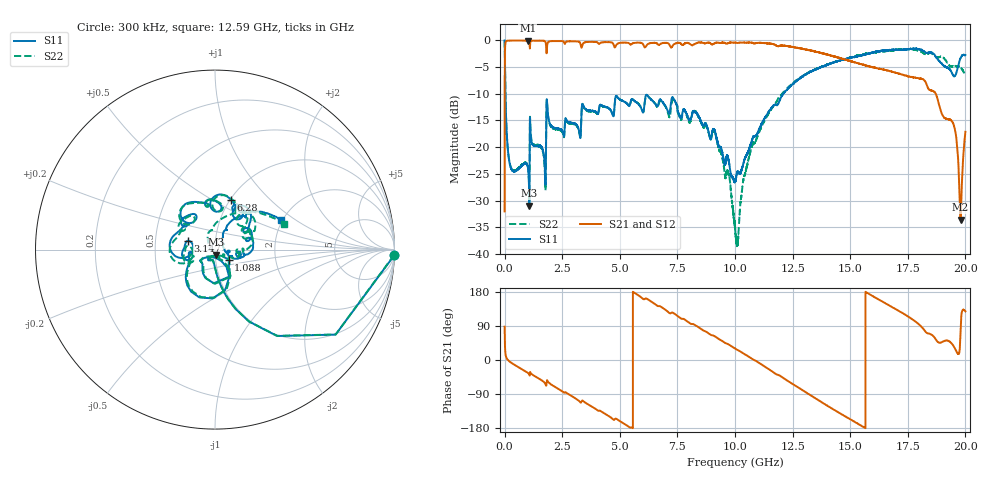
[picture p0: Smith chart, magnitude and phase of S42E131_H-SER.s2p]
! Created Wed Nov 25 21:58:57 2020
# khz S ma R 50
! 2 Port Network Data from SP1.SP block
! freq  magS11  angS11  magS21  angS21  magS12  angS12  magS22  angS22
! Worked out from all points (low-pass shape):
!   20001 points, 300 kHz to 20 GHz, reference 50 ohm
!   highest |S21| = -0.02 dB at 1.005 GHz (marker M1); lowest = -33.6 dB at 19.79 GHz (marker M2)
!   |S21| within 3 dB of the highest: 12.05 MHz to 14.32 GHz (14.3 GHz wide, 200 % of centre); 14.31797 GHz to 14.31964 GHz (1.671 MHz wide, 0.0117 % of centre)
!   lowest |S11| = -31.0 dB at 1.074 GHz (marker M3), VSWR 1.06, Z = 50.4 - j2.82 ohm
!   |S11| at or under -10 dB: 36.14 MHz to 12.1 GHz (12.06 GHz wide, 199 % of centre)
!   |S22| runs from -38.5 to 0.0 dB; largest |S21 - S12| = 0.017
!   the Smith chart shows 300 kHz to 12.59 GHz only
!   S11 on the Smith chart (normalised r, x): 300 kHz: 3, -61; 1.088 GHz: 1.16, -0.13; 3.147 GHz: 0.73, +0.07; 6.28 GHz: 1.01, +0.61; 12.59 GHz: 1.96, +0.78
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300  0.9984 -1.9  0.02499 88.0  0.0251 88.6  0.9984 -1.7
111300  0.1148 -88.3  0.9916 2.4  0.9923 2.4  0.1156 -88.2
323300  0.06085 -100.6  0.9963 -8.7  0.9966 -8.7  0.06155 -99.8
1005300  0.06536 -125.9  0.9975 -33.8  0.9964 -33.7  0.0666 -122.0
1074300  0.02831 -80.8  0.9749 -39.0  0.9755 -39.0  0.03228 -77.2
1088300  0.09454 -36.6  0.902 -41.0  0.9011 -41.0  0.0987 -36.6
3147300  0.1598 162.3  0.9798 -104.0  0.9785 -103.9  0.1569 172.6
3334300  0.202 -166.7  0.855 -110.4  0.8539 -110.4  0.2062 -158.1
4619300  0.2194 118.9  0.9592 -152.1  0.9582 -152.1  0.2184 122.7
6280300  0.2904 71.8  0.9364 157.5  0.9347 157.5  0.2917 69.6
6667300  0.2496 67.4  0.9126 142.2  0.9113 142.1  0.2421 61.7
9111300  0.145 -18.4  0.9353 63.0  0.9389 63.0  0.1388 -13.9
1.00003e7  0.04748 19.6  0.9545 30.4  0.9553 30.4  0.01791 -123.5
1.07373e7  0.116 63.9  0.9504 3.1  0.9503 3.3  0.1019 109.3
1.25883e7  0.4048 24.3  0.8612 -66.6  0.8629 -66.5  0.4105 20.0
1.33343e7  0.5132 -4.3  0.7973 -95.1  0.8017 -94.9  0.5167 -7.1
1.48403e7  0.6744 -64.7  0.657 -150.9  0.6555 -150.9  0.6757 -58.1
1.66673e7  0.8087 -122.9  0.5216 145.2  0.5082 145.4  0.7988 -125.5
1.86843e7  0.7174 154.3  0.324 57.2  0.3238 57.0  0.712 169.5
1.95113e7  0.4613 145.7  0.157 34.1  0.1588 34.1  0.5696 150.2
1.97883e7  0.6781 151.2  0.02092 71.5  0.02069 73.4  0.5531 139.1
2e7  0.7289 134.6  0.1391 128.4  0.1398 129.0  0.476 135.5
